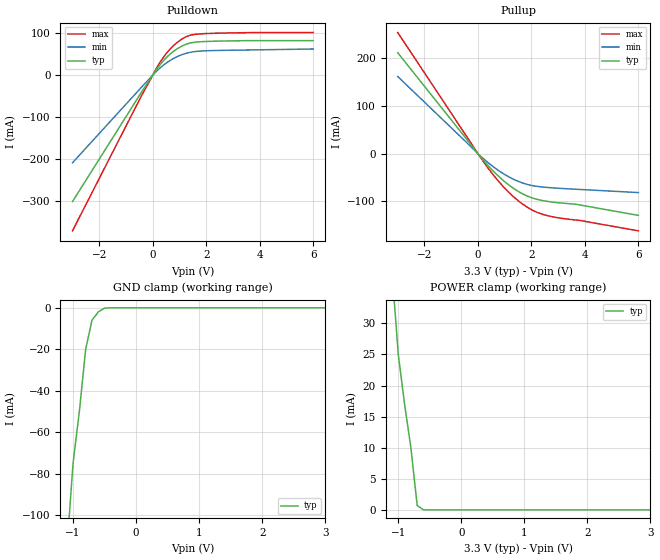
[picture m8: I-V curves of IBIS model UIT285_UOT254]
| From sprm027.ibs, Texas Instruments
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[Model]   UIT285_UOT254
Model_type   I/O
Polarity   Non-Inverting
Enable   Active-Low
| signals   A, GZ, Y
Vinl = 0.8V
Vinh = 2.0V
Cref = 30p
Rref = 50
Vref = 1.5
Vmeas = 1.5
|   typ   min   max
C_comp   4.3750p   4.2590p   4.6039p
|   typ   min   max
[Temperature Range]   25.0   0   90
|   typ   min   max
[Voltage Range]   3.3V   3.13V   3.47V
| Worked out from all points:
|   slope of the pulldown table from 0 to 0.495 V, typ, clamps not added: 12 ohm
|   slope of the pullup table from 0 to 0.495 V, typ, clamps not added: 15.5 ohm
|   GND clamp passes 1 mA (typ) near -0.55 V on its own axis
|   POWER clamp passes 1 mA (typ) near -0.70 V on its own axis
[Pulldown]
|   Voltage   I(typ)   I(min)   I(max)
-3V       -302.4mA   -209.6mA   -372.4mA
-400mV    -38.5mA    -27.34mA   -46.67mA
100mV     9.841mA    6.765mA    12.19mA
300mV     27.11mA    18.76mA    33.55mA
500mV     41.46mA    28.87mA    51.3mA
900mV     62.63mA    44.02mA    77.59mA
1.3V      75.23mA    53.29mA    93.4mA
1.7V      79.7mA     57.38mA    98.5mA
3.9V      82.78mA    60.65mA    102.2mA
6V        82.78mA    62.75mA    102.2mA
[GND_clamp]
|   Voltage   I(typ)   I(min)   I(max)
-3V       -900mA     NA         NA
-2V       -500mA     NA         NA
-1V       -75mA      NA         NA
-900mV    -50mA      NA         NA
-800mV    -20mA      NA         NA
-700mV    -6mA       NA         NA
-600mV    -2mA       NA         NA
-500mV    -120uA     NA         NA
-400mV    0A         NA         NA
3V        0A         NA         NA
[Pullup]
|   Voltage   I(typ)   I(min)   I(max)
-3V       212.1mA    162.1mA    254.5mA
300mV     -20.06mA   -15.17mA   -24.29mA
900mV     -54.01mA   -40.32mA   -66.26mA
1.2V      -67.7mA    -50.15mA   -83.71mA
1.5V      -79.05mA   -58.04mA   -98.65mA
1.8V      -87.95mA   -63.92mA   -110.9mA
2.1V      -94.31mA   -67.74mA   -120.5mA
2.6V      -100.3mA   -71.03mA   -130.3mA
3.7V      -106.7mA   -74.87mA   -139.7mA
6V        -129.7mA   -81.77mA   -162.2mA
[POWER_clamp]
|   Voltage   I(typ)   I(min)   I(max)
-3V       300mA      NA         NA
-2V       160mA      NA         NA
-1V       25mA       NA         NA
-900mV    17mA       NA         NA
-800mV    10mA       NA         NA
-700mV    700uA      NA         NA
-600mV    0A         NA         NA
-500mV    0A         NA         NA
3V        0A         NA         NA
[Ramp]
|   I(typ)   I(min)   I(max)
dV/dt_r   1.570/0.160n   1.331/0.200n   1.732/0.140n
dV/dt_f   1.491/0.170n   1.291/0.220n   1.648/0.130n
